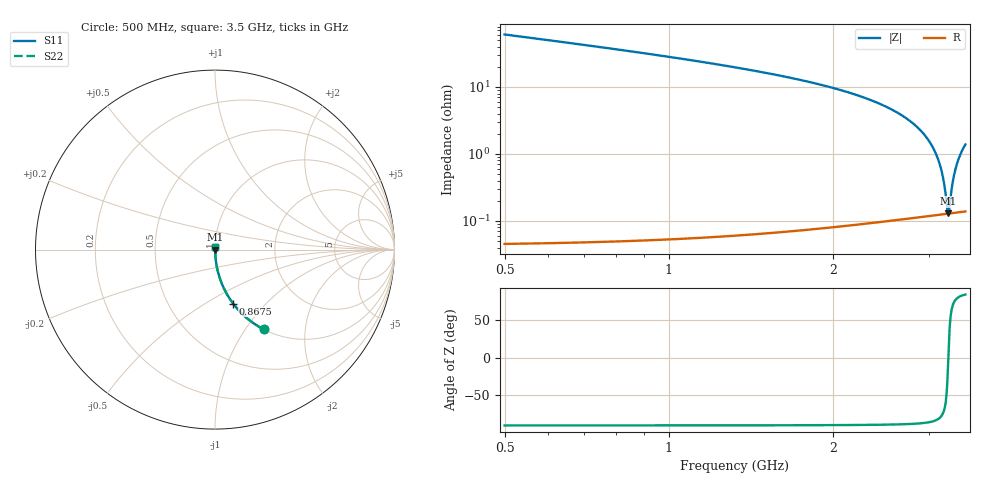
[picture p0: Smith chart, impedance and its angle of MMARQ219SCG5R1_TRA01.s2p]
! MMARQ219SCG5R1_TRA01  S-PARAMETER MODEL  ( General Type )
! Model Generated by TAIYO YUDEN Corporation (http://www.ty-top.com)
! Version 1.0
! TAIYO YUDEN Control No. 180601
! Copyright(c) 2018 TAIYO YUDEN CO.,LTD. All Rights Reserved.
! Product Description (link to TY-COMPAS)
! https://ds.yuden.co.jp/TYCOMPAS/or/detail?pn=MMARQ219SCG5R1CTRA01&u=M
! Products Name : Multilayer Ceramic Capacitors
! Characteristics :
!  Capacitance : 5.1 pF , Rated Voltage : 250V , TCC : CG / C0G
!  Case Size : 2.0 x 1.25 / 0.079 x 0.049 [mm/inch] , Thickness : 0.85 / 0.033 [mm/inch]
!  (Conditions: Temperature = 25 degC , DC Bias Current/Voltage = 0A / 0V)
! External Node Assignments :
!  1  o---| |---o  2
! GND o---------o GND
! Frequency Range : 500MHz  -  3500MHz  [ 401 STEP ]
# MHz S RI R 50
! Freq[MHz].  S11 Real  S11 Imag  S21 Real  S21 Imag  S12 Real  S12 Imag  S22 Real  S22 Imag
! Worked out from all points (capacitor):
!   401 points, 500 MHz to 3.5 GHz, reference 50 ohm
!   read as one part in series: C = 5.1 pF near 515 MHz
!   lowest |Z| = 130 mohm at 3.252 GHz (marker M1)
!   series resonance near 3.256 GHz, so ESL is about 470 pH
!   S11 on the Smith chart (normalised r, x): 500 MHz: 1.00, -1.22; 867.5 MHz: 1.00, -0.67; 3.5 GHz: 1.00, +0.03
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500  0.2712 -0.4442  0.7288 0.4442  0.7288 0.4442  0.2712 -0.4442
665  0.1686 -0.3739  0.8314 0.3739  0.8314 0.3739  0.1686 -0.3739
867.5  0.1009 -0.3004  0.8991 0.3004  0.8991 0.3004  0.1009 -0.3004
1002.5  0.074 -0.2608  0.926 0.2608  0.926 0.2608  0.074 -0.2608
1505  0.0265 -0.1586  0.9735 0.1586  0.9735 0.1586  0.0265 -0.1586
2000  0.0101 -0.096  0.9899 0.096  0.9899 0.096  0.0101 -0.096
2502.5  0.00357 -0.0507  0.9964 0.0507  0.9964 0.0507  0.00357 -0.0507
2802.5  0.00193 -0.0287  0.9981 0.0287  0.9981 0.0287  0.00193 -0.0287
2915  0.00159 -0.0212  0.9984 0.0212  0.9984 0.0212  0.00159 -0.0212
3005  0.00142 -0.0153  0.9986 0.0153  0.9986 0.0153  0.00142 -0.0153
3087.5  0.00132 -0.0102  0.9987 0.0102  0.9987 0.0102  0.00132 -0.0102
3155  0.00128 -0.00603  0.9987 0.00603  0.9987 0.00603  0.00128 -0.00603
3192.5  0.00127 -0.00377  0.9987 0.00377  0.9987 0.00377  0.00127 -0.00377
3215  0.00127 -0.00243  0.9987 0.00243  0.9987 0.00243  0.00127 -0.00243
3237.5  0.00128 -0.0011  0.9987 0.0011  0.9987 0.0011  0.00128 -0.0011
3252.5  0.00128 -0.000222  0.9987 0.000222  0.9987 0.000222  0.00128 -0.000222
3267.5  0.00129 0.000655  0.9987 -0.000655  0.9987 -0.000655  0.00129 0.000655
3312.5  0.00132 0.00326  0.9987 -0.00326  0.9987 -0.00326  0.00132 0.00326
3335  0.00133 0.00455  0.9987 -0.00455  0.9987 -0.00455  0.00133 0.00455
3357.5  0.00136 0.00583  0.9986 -0.00583  0.9986 -0.00583  0.00136 0.00583
3425  0.00144 0.00963  0.9986 -0.00963  0.9986 -0.00963  0.00144 0.00963
3500  0.00157 0.0138  0.9984 -0.0138  0.9984 -0.0138  0.00157 0.0138
